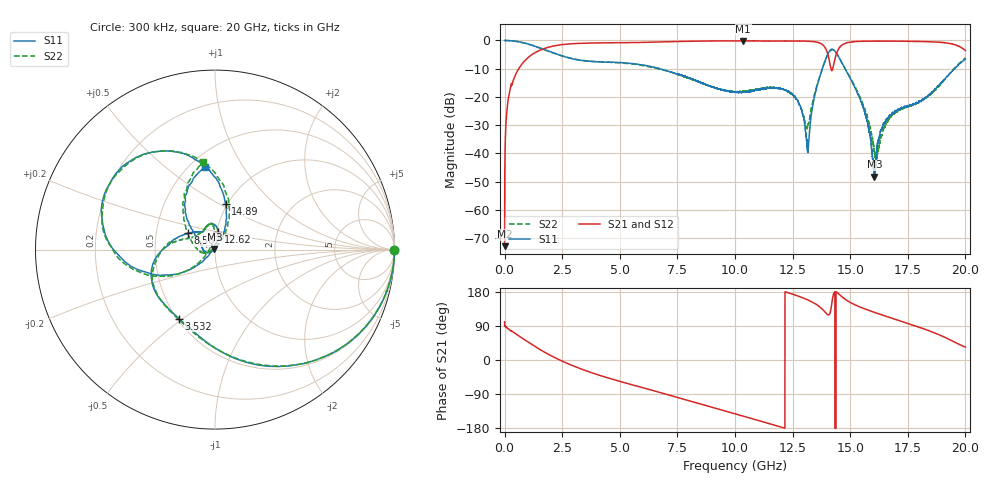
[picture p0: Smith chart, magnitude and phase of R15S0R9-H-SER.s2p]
!{R15S0R9}
!Johanson Technology Inc.
!www.johansontechnology.com
!Test Board Conditions:
!Substrate Type  RO4350B
!Substrate Thickness  20 mil
!Substrate Dk  3.66
!TL Type: GCPW
!TL Trace Width  34 mil
!TL Gap  10 mil
!Electrode orientation  Horizontal
!DUT TOPOLOGY	SERIES
!Mounting Pad LxW  26x52 mil
! Created Sat Feb  6 12:09:23 2021
# hz S ma R 50
! 2 Port Network Data from SP1.SP block
! freq  magS11  angS11  magS21  angS21  magS12  angS12  magS22  angS22
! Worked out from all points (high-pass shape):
!   20001 points, 300 kHz to 20 GHz, reference 50 ohm
!   highest |S21| = -0.14 dB at 10.36 GHz (marker M1); lowest = -72.8 dB at 300 kHz (marker M2)
!   |S21| within 3 dB of the highest: 1.628 GHz to 13.95 GHz (12.32 GHz wide, 158 % of centre); 14.48 GHz to 19.94 GHz (5.454 GHz wide, 31.7 % of centre)
!   lowest |S11| = -48.2 dB at 16.05 GHz (marker M3), VSWR 1.01, Z = 49.7 + j0.174 ohm
!   |S11| at or under -10 dB: 6.732 GHz to 13.79 GHz (7.061 GHz wide, 68.8 % of centre); 14.78 GHz to 19.53 GHz (4.756 GHz wide, 27.7 % of centre)
!   |S22| runs from -42.4 to 0.0 dB; largest |S21 - S12| = 0.013
!   S11 on the Smith chart (normalised r, x): 300 kHz: open; 3.532 GHz: 0.51, -0.48; 8.562 GHz: 0.73, +0.14; 12.62 GHz: 1.01, +0.20; 14.89 GHz: 0.98, +0.53; 20 GHz: 0.59, +0.70
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300000  0.999 -0.1  0.0002286 100.8  0.0001527 112.0  0.9967 -0.2
1.343e8  0.9963 -6.2  0.07754 83.6  0.07796 83.5  0.9967 -6.1
5.193e8  0.9619 -22.0  0.2697 67.7  0.2705 67.8  0.9611 -22.0
1.4753e9  0.7486 -60.3  0.6551 29.7  0.6562 29.6  0.7488 -60.0
3.3343e9  0.4442 -113.3  0.8903 -23.9  0.8919 -23.9  0.4457 -114.1
3.5323e9  0.4342 -117.7  0.8955 -28.3  0.8965 -28.3  0.4357 -118.7
6.6673e9  0.321 -174.5  0.9396 -84.5  0.941 -84.4  0.3147 -174.1
8.5623e9  0.1769 149.2  0.9739 -117.1  0.9763 -117.1  0.1758 160.2
1.00003e10  0.1222 126.9  0.9834 -142.1  0.9831 -142.1  0.1239 131.0
1.03573e10  0.1223 122.7  0.9839 -148.2  0.982 -148.2  0.127 121.7
1.26203e10  0.09863 80.4  0.9745 171.2  0.9729 171.2  0.09592 93.3
1.31373e10  0.0126 127.4  0.9716 159.2  0.9721 159.2  0.02896 158.0
1.33343e10  0.05632 -136.6  0.962 153.6  0.9624 153.6  0.0694 -146.2
1.38603e10  0.3828 -159.2  0.7974 129.8  0.8007 129.1  0.3853 -157.8
1.41263e10  0.6657 162.0  0.3746 123.9  0.3775 123.5  0.6587 162.8
1.43843e10  0.6097 115.8  0.5571 -179.9  0.5554 179.7  0.609 115.6
1.48903e10  0.2592 76.9  0.9128 155.9  0.9134 156.0  0.264 73.2
1.56523e10  0.04959 59.1  0.967 134.4  0.9679 134.7  0.05677 56.0
1.60483e10  0.003892 153.3  0.9723 125.8  0.9726 125.9  0.01093 86.7
1.66673e10  0.04387 -158.6  0.9753 113.0  0.9674 113.2  0.03931 -160.8
1.86543e10  0.1342 144.1  0.9402 71.7  0.9361 71.7  0.1306 163.5
2e10  0.4666 96.3  0.6628 34.1  0.656 34.2  0.4915 97.7
